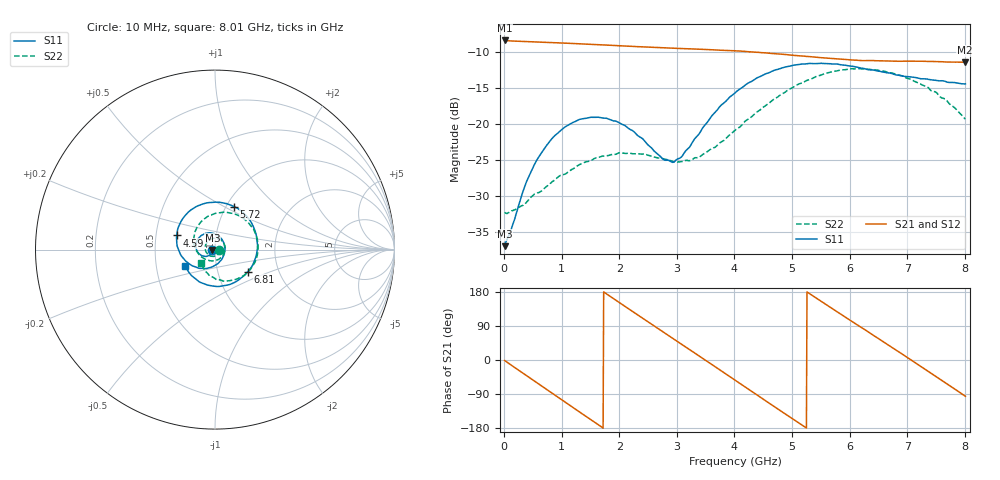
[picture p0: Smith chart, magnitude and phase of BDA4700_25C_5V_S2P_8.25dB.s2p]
!Agilent Technologies,E5071B,MY42404982,A.09.10
!Date: Mon Oct 20 13:30:08 2025
!Data & Calibration Information:
!Freq	S11:SOLT2(ON)	S21:SOLT2(ON)	S12:SOLT2(ON)	S22:SOLT2(ON)
# Hz S RI R 50
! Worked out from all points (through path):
!   801 points, 10 MHz to 8.01 GHz, reference 50 ohm
!   highest |S21| = -8.37 dB at 10 MHz (marker M1); lowest = -11.4 dB at 8 GHz (marker M2)
!   group delay of S21, straight-line fit = 282 ps
!   lowest |S11| = -36.9 dB at 10 MHz (marker M3), VSWR 1.03, Z = 48.6 - j0.159 ohm
!   |S11| at or under -10 dB: start of sweep to end of sweep
!   |S22| runs from -32.4 to -12.3 dB; largest |S21 - S12| = 0.0028
!   S11 on the Smith chart (normalised r, x): 10 MHz: 0.97, -0.00; 4.59 GHz: 0.64, +0.11; 5.72 GHz: 1.09, +0.56; 6.81 GHz: 1.39, -0.36; 8.01 GHz: 0.70, -0.13
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1e7  -0.0142 -0.00164  0.3816 -0.00835  0.3814 -0.00869  0.0245 -0.00132
4e8  -0.0281 -0.0295  0.2767 -0.2528  0.2764 -0.253  0.0186 -0.0224
7.2e8  -0.0585 -0.0375  0.0904 -0.3591  0.0906 -0.3592  -0.00124 -0.0364
1.02e9  -0.0909 -0.021  -0.1069 -0.3501  -0.107 -0.3504  -0.0293 -0.0337
1.35e9  -0.1071 0.0203  -0.2817 -0.2263  -0.2818 -0.2264  -0.053 -0.0048
1.93e9  -0.0559 0.0892  -0.3285 0.1262  -0.3285 0.1265  -0.0233 0.0573
2.32e9  0.00744 0.0831  -0.168 0.3021  -0.168 0.3023  0.0271 0.0563
2.68e9  0.0491 0.0372  0.0448 0.338  0.0447 0.3378  0.0558 0.0171
2.96e9  0.0527 -0.016  0.1981 0.2725  0.1982 0.2721  0.051 -0.0198
3.37e9  0.00647 -0.0838  0.3244 0.0704  0.3249 0.0704  0.00916 -0.058
3.68e9  -0.0634 -0.1052  0.3092 -0.1084  0.3094 -0.1094  -0.0373 -0.0591
4.01e9  -0.1453 -0.0782  0.1941 -0.2587  0.1945 -0.2585  -0.0844 -0.0332
4.59e9  -0.2133 0.0788  -0.1196 -0.2878  -0.1192 -0.2882  -0.1159 0.0772
4.99e9  -0.1536 0.2036  -0.2694 -0.1362  -0.27 -0.1366  -0.0672 0.1652
5.35e9  -0.0349 0.2617  -0.2895 0.0488  -0.2898 0.0481  0.0289 0.2057
5.72e9  0.1071 0.2391  -0.1966 0.207  -0.1964 0.2074  0.1431 0.1833
6.18e9  0.2223 0.1057  0.00908 0.2771  0.0108 0.2777  0.2344 0.0628
6.68e9  0.2114 -0.0828  0.2147 0.1716  0.2153 0.1713  0.2091 -0.092
6.81e9  0.1818 -0.1235  0.247 0.119  0.2477 0.1179  0.1847 -0.1219
7.33e9  0.0162 -0.2057  0.2445 -0.1219  0.2448 -0.1226  0.0506 -0.176
8e9  -0.1662 -0.0936  -0.0221 -0.2683  -0.0221 -0.2688  -0.0751 -0.0798
8.01e9  -0.168 -0.0908  -0.0271 -0.2679  -0.0266 -0.2682  -0.0759 -0.0774
